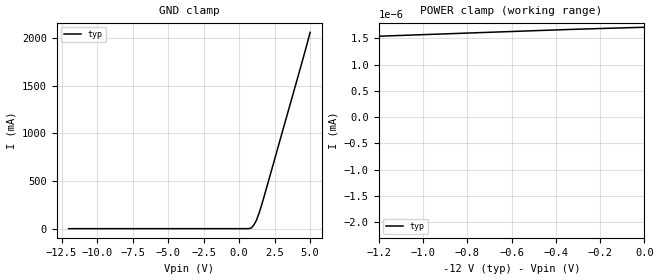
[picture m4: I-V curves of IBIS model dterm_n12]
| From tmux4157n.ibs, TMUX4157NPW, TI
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| dterm_n12
[Model]   dterm_n12
Model_type   Terminator
|   typ   min   max
C_comp   1.008417e-11   NA   NA
[Voltage Range]   -12   NA   NA
[Temperature Range]   27   NA   NA
[Power Clamp Reference]   -12   NA   NA
[GND Clamp Reference]   0   NA   NA
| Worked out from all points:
|   POWER clamp passes 1 mA (typ) near -12.71 V on its own axis
[GND Clamp]
|   Voltage   I(typ)   I(min)   I(max)
-12V      -1.458nA   NA         NA
535.4mV   23.31uA    NA         NA
878.8mV   9.52mA     NA         NA
1.051V    41.39mA    NA         NA
1.222V    88.25mA    NA         NA
1.566V    237.6mA    NA         NA
4.313V    1.685A     NA         NA
5V        2.06A      NA         NA
[POWER Clamp]
|   Voltage   I(typ)   I(min)   I(max)
-17V      -2.159A    NA         NA
-12.19V   -2.226nA   NA         NA
-12.02V   -1.464nA   NA         NA
-10.3V    -961.8pA   NA         NA
-7.899V   -360.6pA   NA         NA
-7.384V   -201.8pA   NA         NA
-7.04V    -5.727pA   NA         NA
-6.869V   160.8pA    NA         NA
-6.525V   577.9pA    NA         NA
-6.354V   644.4pA    NA         NA
-3.778V   1.129nA    NA         NA
0V        1.709nA    NA         NA
